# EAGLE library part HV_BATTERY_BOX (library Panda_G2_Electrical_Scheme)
HV battery box
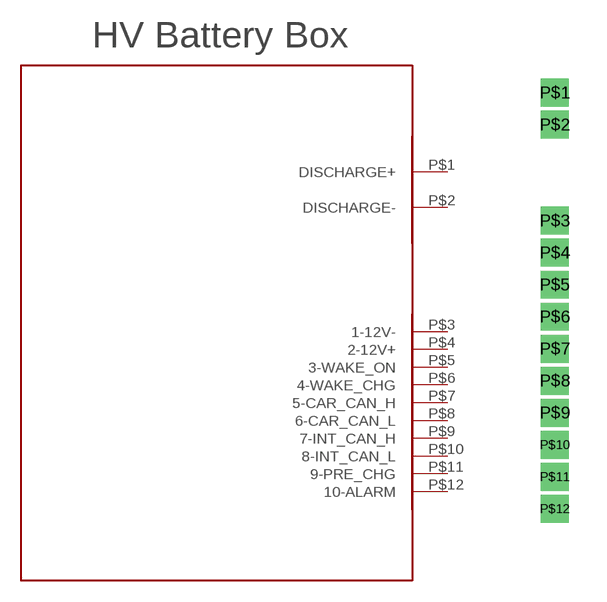
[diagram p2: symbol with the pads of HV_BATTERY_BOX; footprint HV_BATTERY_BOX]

Designator prefix -

## HV_BATTERY_BOX  [HV_BATTERY_BOX]
P$1  DISCHARGE+  pwr
P$2  DISCHARGE-  pwr
P$3  1-12V-
P$4  2-12V+
P$5  3-WAKE_ON
P$6  4-WAKE_CHG
P$7  5-CAR_CAN_H
P$8  6-CAR_CAN_L
P$9  7-INT_CAN_H
P$10  8-INT_CAN_L
P$11  9-PRE_CHG
P$12  10-ALARM

## Footprint HV_BATTERY_BOX (pad centres in mm)
drill 0.6 square: P$1 0,17.78; P$2 0,16.51; P$3 0,12.7; P$4 0,11.43; P$5 0,10.16; P$6 0,8.89; P$7 0,7.62; P$8 0,6.35; P$9 0,5.08; P$10 0,3.81; P$11 0,2.54; P$12 0,1.27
